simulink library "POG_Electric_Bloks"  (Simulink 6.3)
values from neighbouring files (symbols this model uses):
  al = Tipo(2)    [Flusso_Rotorico_An.m]
  bm = 0.8*N*metri*secondo/rad    (= 0.8)    [architetture_epicicloidale.m]    (also in architetture_epicicloidale_cont.m; architetture_epicicloidale_HEV.m; architetture_epicicloidale_prova.m; architetture_HEV_controllo.m)
  Iw0 = 0*wI0    [architetture_epicicloidale.m]    (also in architetture_epicicloidale_cont.m = wI0; architetture_epicicloidale_HEV.m; architetture_epicicloidale_prova.m; architetture_HEV_controllo.m)
  Jm = 1.6*kg*metri^2    (= 1.6)    [architetture_epicicloidale.m]    (also in architetture_epicicloidale_cont.m; architetture_epicicloidale_HEV.m = 1.64945909552; architetture_epicicloidale_prova.m; architetture_HEV_controllo.m = 0.529459095518)
  Li = 0.1*Henry    (= 0.1)    [architetture_epicicloidale.m]    (also in architetture_epicicloidale_cont.m; architetture_epicicloidale_HEV.m; architetture_epicicloidale_prova.m; architetture_HEV_controllo.m)
  m = 5    [architetture_epicicloidale.m]    (also in architetture_epicicloidale_cont.m; architetture_epicicloidale_HEV.m; architetture_epicicloidale_prova.m; architetture_HEV_controllo.m)
  Mi = 0.08*Henry    (= 0.08)    [architetture_epicicloidale.m]    (also in architetture_epicicloidale_cont.m; architetture_epicicloidale_HEV.m; architetture_epicicloidale_prova.m; architetture_HEV_controllo.m)
  ms = 0.001*secondo    (= 0.001)    [architetture_epicicloidale.m]    (also in architetture_epicicloidale_cont.m; architetture_epicicloidale_HEV.m; architetture_epicicloidale_prova.m; architetture_HEV_controllo.m)
  Nar = 200    [architetture_epicicloidale.m]    (also in architetture_epicicloidale_cont.m; architetture_epicicloidale_HEV.m; architetture_epicicloidale_prova.m; architetture_HEV_controllo.m)
  Nc = 30    [architetture_epicicloidale.m]    (also in architetture_epicicloidale_cont.m; architetture_epicicloidale_HEV.m; architetture_epicicloidale_prova.m; architetture_HEV_controllo.m)
  p = 1    [architetture_epicicloidale.m]    (also in architetture_epicicloidale_cont.m; architetture_epicicloidale_HEV.m; architetture_epicicloidale_prova.m; architetture_HEV_controllo.m)
  Phir = 0.02*Weber    (= 0.02)    [architetture_epicicloidale.m]    (also in architetture_epicicloidale_cont.m; architetture_epicicloidale_HEV.m; architetture_epicicloidale_prova.m; architetture_HEV_controllo.m)
  Ri = 3*Ohm    (= 3)    [architetture_epicicloidale.m]    (also in architetture_epicicloidale_cont.m; architetture_epicicloidale_HEV.m; architetture_epicicloidale_prova.m; architetture_HEV_controllo.m = 0.1)
  Rr = 0.905*m    (= 0.905)    [CVT_New.m]    (also in CVT_New_th.m)
  Star = Si    [architetture_epicicloidale.m]    (also in architetture_epicicloidale_cont.m; architetture_epicicloidale_HEV.m; architetture_epicicloidale_prova.m; architetture_HEV_controllo.m)
  Thm0 = 0    [architetture_epicicloidale.m]    (also in architetture_epicicloidale_cont.m; architetture_epicicloidale_HEV.m; architetture_epicicloidale_prova.m; architetture_HEV_controllo.m)
  Tipo = eval(Flusso(ij).Tipo)    [architetture_epicicloidale.m]    (also in architetture_epicicloidale_cont.m; architetture_epicicloidale_HEV.m; architetture_epicicloidale_prova.m; architetture_HEV_controllo.m)
  Wm0 = 0*Wr_d    (= 0)    [architetture_epicicloidale.m]    (also in architetture_epicicloidale_cont.m = 62.5; architetture_epicicloidale_HEV.m; architetture_epicicloidale_prova.m; architetture_HEV_controllo.m)
undefined symbols (not defined in the file or in its folder): Ib0, Lr, Ls, Lwe, mr, Mr0, Ms0, Msr0, Rs, Rwe
libraries: simulink x10
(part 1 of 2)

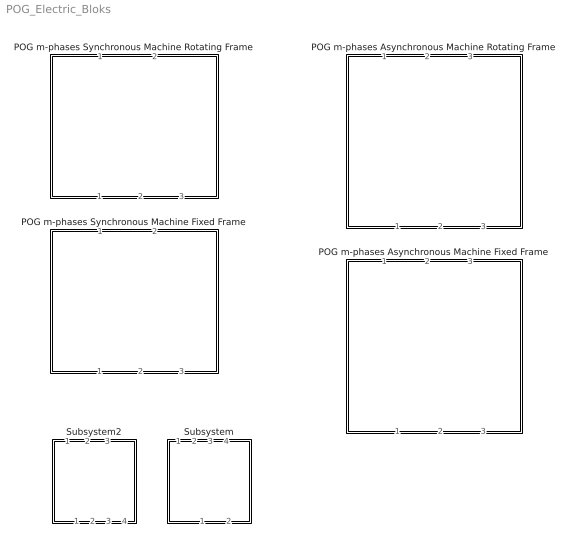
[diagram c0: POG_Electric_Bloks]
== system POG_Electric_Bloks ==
  POG m-phases Asynchronous Machine Fixed Frame : Subsystem  Orientation=down  mask(POG Multi-Phase Motor (Rotating Frame)){Motor_Par=[ms mr], Polar_Par=[p], Electric_S_Par=[Ls Ms0 Rs], Electric_R_Par=[Lr Mr0 Rr], Msr0=Msr0, Mech_Par=[Jm bm], Iniz_Cond=[Wm0; Thm0; Ib0]}
      mask prompts: Motor_Par "Number of phases: [ms, mr] -> [Nr, Nr]"; Polar_Par "Number of polar couples: [p] -> [Nr]"; Electric_S_Par "Stator Parameters: [Ls, Ms0, Rs] -> [Henry, Henry, Ohm]"; Electric_R_Par "Rotor Parameters: [Lr, Mr0, Rr] -> [Henry, Henry, Ohm]"; Msr0 "Mutual Inductance coefficient: [Msr0]-> [Henry]"; Mech_Par "Mechanical Parameters: [Jm, bm] -> [kg*m^2, N m s/rad]"; Iniz_Cond "Initial conditions: [Wm0, Thm0, Ib0] -> [rad/s, rad, A]"
      mask help: Multi-Phase Asynchronous Motor: [ms,mr] = Number of stator and rotor phases; [p] = Number of polar couples; [Ls, Ms0, Rs] = Self inductance, Mutual inductance and Resistance of each stator phase (p=1); [Lr, Mr0, Rr] = Self inductance, Mutual inductance and Resistance of each rotor phase (p=1); [Msr0] = Mutual Inductance coefficient; [Jm, bm] = Inertia momentum, Linear friction coefficient of the rotor; [Wm0, Thm0, Iw0] = Initial conditions on Velocity, Position of the motor and Transformed currents;
      mask init:
      | ms=Motor_Par(1);
      | mr=Motor_Par(2);
      | p =Polar_Par(1);
      | Ls =Electric_S_Par(1);
      | Ms0=Electric_S_Par(2);
      | Rs =Electric_S_Par(3);
      | Lr =Electric_R_Par(1);
      | Mr0=Electric_R_Par(2);
      | Rr =Electric_R_Par(3);
      | Jm=Mech_Par(1);
      | bm=Mech_Par(2);
      | 
      | %%%%%%%%%%%%%%%%%%%%% Initial Conditions
      | if length(Iniz_Cond)<(ms+mr)
      |     Iniz_Cond=[Iniz_Cond; 0*[1:ms+mr-length(Iniz_Cond)]'];
      |     disp('Correction: Iniz_Cond = ...');
      |     disp(Iniz_Cond)
      | end
      | Wm0 = Iniz_Cond(1);
      | Thm0= Iniz_Cond(2);
      | Ib0 = Iniz_Cond(3:ms+mr);
      | 
      | %%%%%%%%%%%%%%%%%%%%%%%%%%%%%%%%%%%%%%%%%%%%%%%%%%%%%%%%%%%%%%%%%%
      | 
      | Ls0=Ls-Ms0;             % stator dispersion self inductance coefficient (p=1)
      | Lse=Ls+(ms-2)*Ms0/2;    % stator transformed self inductance coefficient (p=1)
      | 
      | Lr0=Lr-Mr0;             % rotor dispersion self inductance coefficient (p=1)
      | Lre=Lr+(mr-2)*Mr0/2;    % rotor transformed self inductance coefficient (p=1)
      | 
      | Msre=Msr0*sqrt(ms*mr)/2; % stator-rotor transformed mutual inductance coefficient (p=1)
      | 
      | %%%%%%%%%%%%%%%%%%%%%%%%%%%%%%%%%%%%%%%%%%%%%%%%%%%%%%%%%%%%%%%%%%
      | %%%%%% Trasformazione di coordinate T(s->t)
      | %%%%%%%%%%%%%%%%%%%%%%%%%%%%%%%%%%%%%%%%%%%%%%%%%%%%%%%%%%%%%%%%%%
      | 
      | sTt=[eye(ms) zeros(ms,mr)];
      | 
      | %%%%%%%%%%%%%%%%%%%%%%%%%%%%%%%%%%%%%%%%%%%%%%%%%%%%%%%%%%%%%%%%%%
      | %%%%%% Trasformazione di coordinate T(t->b)
      | %%%%%%%%%%%%%%%%%%%%%%%%%%%%%%%%%%%%%%%%%%%%%%%%%%%%%%%%%%%%%%%%%%
      | 
      | tTb=zeros(ms+mr,ms+mr-2);   
      | %
      | %%%%%%%%%%%%%%%%%%%%%%%%%%%%%%%%%%%%%%%%%%%%%%
      | T_b_Concordia = zeros(ms,ms-1);
      | w = 2*pi/ms;
      | for ii = [1:ms/2]
      |     for jj = [0:ms-1]
      |         T_b_Concordia(jj+1,2*ii-1) = cos((2*ii-1)*w*jj);
      |         T_b_Concordia(jj+1,2*ii  ) = sin((2*ii-1)*w*jj);
      |     end
      | end
      | tTb(1:ms,1:ms-1)=sqrt(2/ms)*T_b_Concordia;       
      | %
      | %%%%%%%%%%%%%%%%%%%%%%%%%%%%%%%%%%%%%%%%%%%%%%
      | T_b_Concordia = zeros(mr,mr-1);
      | w = 2*pi/mr;
      | for ii = [1:mr/2]
      |     for jj = [0:mr-1]
      |         T_b_Concordia(jj+1,2*ii-1) = cos((2*ii-1)*w*jj);
      |         T_b_Concordia(jj+1,2*ii  ) = sin((2*ii-1)*w*jj);
      |     end
      | end
      | tTb(ms+1:ms+mr,ms:ms+mr-2)=sqrt(2/mr)*T_b_Concordia;       
      | 
      | %%%%%%%%%%%%%%%%%%%%%%%%%%%%%%%%%%%%%%%%%%%%%%%%%%%%%%%%%%%%%%%%%%
      | %%%%%% Matrici LMbe e Rbe nel frame ruotante w
      | %%%%%%%%%%%%%%%%%%%%%%%%%%%%%%%%%%%%%%%%%%%%%%%%%%%%%%%%%%%%%%%%%%
      | 
      | LMbe=zeros(ms+mr-2);            % Matrice LMbe
      | LMbe(1:2,1:2)=eye(2)*Lse;        
      | LMbe(3:ms-1,3:ms-1)=eye(ms-3)*Ls0;        
      | LMbe(ms:ms+1,ms:ms+1)=eye(2)*Lre;        
      | LMbe(ms+2:ms+mr-2,ms+2:ms+mr-2)=eye(mr-3)*Lr0;        
      | LMbe=p*LMbe;
      | 
      | Mbe=zeros(ms+mr-2);            % Matrice Mbe
      | Mbe(1:2,ms:ms+1)=eye(2);        
      | Mbe(ms:ms+1,1:2)=eye(2);        
      | 
      | JKb=zeros(ms+mr-2);            % Matrice JKb             
      | JKb(2,1)=-1;  
      | JKb(1,2)=1;  
      | JKb(ms+1,ms)=1;  
      | JKb(ms,ms+1)=-1;  
      | 
      | Lbe=LMbe+Mbe*cos(p*Thm0)-JKb*sin(p*Thm0);
      | 
      | Rbe=zeros(ms+mr-2);            % Matrice Rbe
      | Rbe(1:ms-1,1:ms-1)=eye(ms-1)*Rs;        
      | Rbe(ms:ms+mr-2,ms:ms+mr-2)=eye(mr-1)*Rr;        
      | 
      | %%%%%%%%%%%%%%%%%%%%%%%%%%%%%%%%%%%%%%%%%%%%%%%%%%%%%%%%%%%%%%%%%%
  POG m-phases Asynchronous Machine Rotating Frame : Subsystem  Orientation=down  mask(POG Multi-Phase Motor (Rotating Frame)){Motor_Par=[ms mr], Polar_Par=[p], Electric_S_Par=[Ls Ms0 Rs], Electric_R_Par=[Lr Mr0 Rr], Msr0=Msr0, Mech_Par=[Jm bm], Iniz_Cond=[Wm0; Thm0; Iw0]}
      mask prompts: Motor_Par "Number of phases: [ms, mr] -> [Nr, Nr]"; Polar_Par "Number of polar couples: [p] -> [Nr]"; Electric_S_Par "Stator Parameters: [Ls, Ms0, Rs] -> [Henry, Henry, Ohm]"; Electric_R_Par "Rotor Parameters: [Lr, Mr0, Rr] -> [Henry, Henry, Ohm]"; Msr0 "Mutual Inductance coefficient: [Msr0]-> [Henry]"; Mech_Par "Mechanical Parameters: [Jm, bm] -> [kg*m^2, N m s/rad]"; Iniz_Cond "Initial conditions: [Wm0, Thm0, Iw0] -> [rad/s, rad, A]"
      mask help: Multi-Phase Asynchronous Motor: [ms,mr] = Number of stator and rotor phases; [p] = Number of polar couples; [Ls, Ms0, Rs] = Self inductance, Mutual inductance and Resistance of each stator phase (p=1); [Lr, Mr0, Rr] = Self inductance, Mutual inductance and Resistance of each rotor phase (p=1); [Msr0] = Mutual Inductance coefficient; [Jm, bm] = Inertia momentum, Linear friction coefficient of the rotor; [Wm0, Thm0, Iw0] = Initial conditions on Velocity, Position of the motor and Transformed currents;
      mask init:
      | ms=Motor_Par(1);
      | mr=Motor_Par(2);
      | p =Polar_Par(1);
      | Ls =Electric_S_Par(1);
      | Ms0=Electric_S_Par(2);
      | Rs =Electric_S_Par(3);
      | Lr =Electric_R_Par(1);
      | Mr0=Electric_R_Par(2);
      | Rr =Electric_R_Par(3);
      | Jm=Mech_Par(1);
      | bm=Mech_Par(2);
      | 
      | %%%%%%%%%%%%%%%%%%%%% Initial Conditions
      | if length(Iniz_Cond)<(ms+mr)
      |     Iniz_Cond=[Iniz_Cond; 0*[1:ms+mr-length(Iniz_Cond)]'];
      |     disp('Correction: Iniz_Cond = ...');
      |     disp(Iniz_Cond)
      | end
      | Wm0 = Iniz_Cond(1);
      | Thm0= Iniz_Cond(2);
      | Iw0 = Iniz_Cond(3:ms+mr);
      | 
      | Ls0=Ls-Ms0;             % stator dispersion self inductance coefficient (p=1)
      | Lse=Ls+(ms-2)*Ms0/2;    % stator transformed self inductance coefficient (p=1)
      | 
      | Lr0=Lr-Mr0;             % rotor dispersion self inductance coefficient (p=1)
      | Lre=Lr+(mr-2)*Mr0/2;    % rotor transformed self inductance coefficient (p=1)
      | 
      | Msre=Msr0*sqrt(ms*mr)/2; % stator-rotor transformed mutual inductance coefficient (p=1)
      | 
      | %%%%%%%%%%%%%%%%%%%%%%%%%%%%%%%%%%%%%%%%%%%%%%%%%%%%%%%%%%%%%%%%%%
      | %%%%%% Trasformazione di coordinate T(s->t)
      | %%%%%%%%%%%%%%%%%%%%%%%%%%%%%%%%%%%%%%%%%%%%%%%%%%%%%%%%%%%%%%%%%%
      | 
      | sTt=[eye(ms) zeros(ms,mr)];
      | 
      | %%%%%%%%%%%%%%%%%%%%%%%%%%%%%%%%%%%%%%%%%%%%%%%%%%%%%%%%%%%%%%%%%%
      | %%%%%% Trasformazione di coordinate T(t->b)
      | %%%%%%%%%%%%%%%%%%%%%%%%%%%%%%%%%%%%%%%%%%%%%%%%%%%%%%%%%%%%%%%%%%
      | 
      | tTb=zeros(ms+mr,ms+mr-2);   
      | %
      | %%%%%%%%%%%%%%%%%%%%%%%%%%%%%%%%%%%%%%%%%%%%%%
      | T_b_Concordia = zeros(ms,ms-1);
      | w = 2*pi/ms;
      | for i = [1:ms/2]
      |     for j = [0:ms-1]
      |         T_b_Concordia(j+1,2*i-1) = cos((2*i-1)*w*j);
      |         T_b_Concordia(j+1,2*i  ) = sin((2*i-1)*w*j);
      |     end
      | end
      | tTb(1:ms,1:ms-1)=sqrt(2/ms)*T_b_Concordia;       
      | %
      | %%%%%%%%%%%%%%%%%%%%%%%%%%%%%%%%%%%%%%%%%%%%%%
      | T_b_Concordia = zeros(mr,mr-1);
      | w = 2*pi/mr;
      | for i = [1:mr/2]
      |     for j = [0:mr-1]
      |         T_b_Concordia(j+1,2*i-1) = cos((2*i-1)*w*j);
      |         T_b_Concordia(j+1,2*i  ) = sin((2*i-1)*w*j);
      |     end
      | end
      | tTb(ms+1:ms+mr,ms:ms+mr-2)=sqrt(2/mr)*T_b_Concordia;       
      | 
      | %%%%%%%%%%%%%%%%%%%%%%%%%%%%%%%%%%%%%%%%%%%%%%%%%%%%%%%%%%%%%%%%%%
      | %%%%%% Trasformazione di coordinate T(b->w)
      | %%%%%%%%%%%%%%%%%%%%%%%%%%%%%%%%%%%%%%%%%%%%%%%%%%%%%%%%%%%%%%%%%%
      | 
      | MKs=zeros(ms+mr-2);             % Matrice MKs
      | MKs(1:2,1:2)=eye(2);  
      | 
      | MKr=zeros(ms+mr-2);             % Matrice MKr             
      | MKr(ms:ms+1,ms:ms+1)=eye(2);  
      | 
      | I_m=eye(ms+mr-2);               % Matrice I_m
      | 
      | Jsr= zeros(ms+mr-2);            % Matrice Jsr
      | for j=[2:2:ms+mr-2]
      |     Jsr(j,j-1)= 1;
      |     Jsr(j-1,j)=-1;
      | end
      | 
      | %%%%%%%%%%%%%%%%%%%%%%%%%%%%%%%%%%%%%%%%%%%%%%%%%%%%%%%%%%%%%%%%%%
      | %%%%%% Matrici Lw_e e Rw_e nel frame ruotante w
      | %%%%%%%%%%%%%%%%%%%%%%%%%%%%%%%%%%%%%%%%%%%%%%%%%%%%%%%%%%%%%%%%%%
      | 
      | Lwe=zeros(ms+mr-2);            % Matrice Lw_e
      | Lwe(1:2,1:2)=eye(2)*Lse;        
      | Lwe(3:ms-1,3:ms-1)=eye(ms-3)*Ls0;        
      | Lwe(ms:ms+1,ms:ms+1)=eye(2)*Lre;        
      | Lwe(ms+2:ms+mr-2,ms+2:ms+mr-2)=eye(mr-3)*Lr0;        
      | Lwe(1:2,ms:ms+1)=eye(2)*Msre;        
      | Lwe(ms:ms+1,1:2)=eye(2)*Msre;        
      | Lwe=p*Lwe;
      | 
      | 
      | Rwe=zeros(ms+mr-2);            % Matrice Rw_e
      | Rwe(1:ms-1,1:ms-1)=eye(ms-1)*Rs;        
      | Rwe(ms:ms+mr-2,ms:ms+mr-2)=eye(mr-1)*Rr;        
      | 
      | Ks=zeros(ms+mr-2,1);           % Matrice Ks
      | Ks(1:2)=[1;1];  
      | 
      | Kr=zeros(ms+mr-2,1);           % Matrice Kr             
      | Kr(ms:ms+1)=[1;1];  
      | 
      | JK=zeros(ms+mr-2);            % Matrice JKe             
      | JK(ms+1,1)=1;  
      | JK(ms,2)=-1;  
      | JK(1,ms+1)=1;  
      | JK(2,ms)=-1;  
      | JKe=-p^2*Msre*JK/2;
      | JFe=p*Msre*JK/2;
      | 
      | %%%%%%%%%%%%%%%%%%%%%%%%%%%%%%%%%%%%%%%%%%%%%%%%%%%%%%%%%%%%%%%%%%
  POG m-phases Synchronous Machine Fixed Frame : Subsystem  Orientation=down  mask(POG Multi-Phase Motor (Fixed Frame)){Motor_Par=[m p], Phase_Par=[Nc Star], Electric_Par=[Ri Li Mi], Mech_Par=[Jm bm], Plux_Par=[Phir Nar], Iniz_Cond=[Wm0; Thm0; Iw0], TipoFlux=Fourier defined, Tipo=Tipo, alfa=al, degree=6, TipoF=Tipo}
      mask prompts: Motor_Par "Number of phases, Number of polar couples: [m, p] -> [Nr, Nr]"; Phase_Par "Number of coils, Star connected?: [Nc, Star] -> [Nr, (True, False)]"; Electric_Par "Electric Parameters: [Ri, Li, Mi] -> [Henry, Henry, Ohm]"; Mech_Par "Mechanical Parameters: [Jm, bm] -> [kg*m^2, N m s/rad]"; Plux_Par "Maximum value of the rotor flux, Number of Fourier harmonics: [Phir, Nar] -> [W, Nr]"; Iniz_Cond "Initial conditions: [Wm0, Thm0, It0] -> [rad/s, rad, A]"; TipoFlux "Type of Rotor Flux"; Tipo "Type defined by user: Tipo -> [Nr,alfa,degree]"; alfa "Flux function parameter: alfa -> [0, pi/2]:"; degree "Degree of the polinomial flux function:"; TipoF "Components of the Fourier series: [9, Nmax, CompAi] -> [9, Nr, a0, a1, ..., aNr]"
      mask help: Multi-Phase Permanent Magnet Synchronous Motor: [m, p] = Number of motor phases, Polar couples; [Nc, Star] = Number of coils per phase, Type of phase connection; [Ri, Li, Mi] = Resistance, Self inductance, Mutual inductance of each phase; [Jm, bm] = Inertia momentum, Friction coefficient of the rotor; [Phir, Nar] = Maximum value of the rotor flux, Number of Fourier harmonics; [Wm0, Thm0, Iw0] = Initial conditions on Velocity, Position of the motor and Currents; Type of Rotor Flux (Tipo): Trapezoidal [1,alfa]; Triangular [1, 0]; Squared wave [2]; Sinusoidal [3]; Cosinusoidally connected [4,alfa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
      mask init:
      | m=Motor_Par(1);
      | p=Motor_Par(2);
      | Nc=Phase_Par(1);
      | Star=Phase_Par(2);
      | Ri=Electric_Par(1);
      | Li=Electric_Par(2);
      | Mi=Electric_Par(3);
      | Jm=Mech_Par(1);
      | bm=Mech_Par(2);
      | Phir=Plux_Par(1);
      | Nar=Plux_Par(2);
      | 
      | %%%%%%%%%%%%%%%%%%%%% Initial Conditions
      | if length(Iniz_Cond)<(m+2-Star)
      |     Iniz_Cond=[Iniz_Cond 0*[1:m+2-Star-length(Iniz_Cond)]];
      |     disp('Correction: Iniz_Cond = ...');
      |     disp(Iniz_Cond)
      | end
      | Wm0 = Iniz_Cond(1);
      | Thm0= Iniz_Cond(2);
      | Ibt0 = Iniz_Cond(3:m+2-Star);
      | 
      | %%%%%%%%%%%%%%%%%%%%%%%%%%%%
      | FluxName(1)=struct('Nome','Trapezoidal');
      | FluxName(2)=struct('Nome','Squared wave');
      | FluxName(3)=struct('Nome','Sinusoidal');
      | FluxName(4)=struct('Nome','Cosinusoidally connected');
      | FluxName(5)=struct('Nome','Sinusoidally connected');
      | FluxName(6)=struct('Nome','Polynomial even');
      | FluxName(7)=struct('Nome','Polynomial odd');
      | FluxName(8)=struct('Nome','Trapezoidal if derived');
      | FluxName(9)=struct('Nome','Fourier defined');
      | 
      | switch TipoFlux
      |     case 'User defined',
      |     case 'Trapezoidal'
      |         if alfa<0, alfa=0; disp('Correction: alfa = 0'); end
      |         if alfa>pi/2, alfa=pi/2; disp('Correction: alfa = pi/2'); end
      |         Tipo = [1,alfa];
      |     case 'Triangular'
      |         Tipo = [1,  0];
      |     case 'Squared wave'
      |         Tipo = [2];
      |     case 'Sinusoidal'
      |         Tipo = [3];
      |     case 'Cosinusoidally connected'
      |         if alfa<0, alfa=0; disp('Correction: alfa = 0'); end
      |         if alfa>pi/2, alfa=pi/2; disp('Correction: alfa = pi/2'); end
      |         Tipo = [4,alfa];
      |     case 'Sinusoidally connected'
      |         if alfa<0, alfa=0; disp('Correction: alfa = 0'); end
      |         if alfa>pi/2, alfa=pi/2; disp('Correction: alfa = pi/2'); end
      |         Tipo = [5,alfa];
      |     case 'Polynomial even'
      |         if alfa<0, alfa=0; disp('Correction: alfa = 0'); end
      |         if alfa>pi/2, alfa=pi/2; disp('Correction: alfa = pi/2'); end
      |         if rem(degree)==1, 
      |             degree=degree-1; 
      |             disp(['Correction: degree = ' num2str(degree)]); 
      |         end
      |         if degree<2
      |             degree=2; 
      |             disp(['Correction: degree = ' num2str(degree)]); 
      |         end            
      |         Tipo = [6,alfa,degree];
      |     case 'Polynomial odd'
      |         if alfa<0, alfa=0; disp('Correction: alfa = 0'); end
      |         if alfa>pi/2, alfa=pi/2; disp('Correction: alfa = pi/2'); end
      |         if rem(degree)==0, 
      |             degree=degree-1; 
      |             disp(['Correction: degree = ' num2str(degree)]); 
      |         end
      |         if degree<1
      |             degree=1; 
      |             disp(['Correction: degree = ' num2str(degree)]); 
      |         end            
      |         Tipo = [7,alfa,degree];
      |     case 'Trapezoidal if derived'
      |         Tipo = [8,alfa];
      |         if alfa<0, alfa=0; disp('Correction: alfa = 0'); end
      |         if alfa>pi/2, alfa=pi/2; disp('Correction: alfa = pi/2'); end
      |     case 'Fourier defined'
      |         if TipoF(1)~=9
      |             disp('Correction: NrType = 9 (Fourier defined)')
      |             TipoF(1)=9;
      |         end
      |         if length(TipoF)<2
      |             TipoF(2)=m;
      |             disp('Correction: Fourier defined -> TipoF = ...');
      |             disp(TipoF)
      |         end
      |         if TipoF(2)<m,
      |             TipoF(2)=m;
      |             disp('Correction: Fourier defined -> Nas = m');
      |         end
      |         if length(TipoF)<(TipoF(2)+3)
      |             TipoF=[TipoF 0*[1:TipoF(2)+3-length(TipoF)]];
      |             disp('Correction: Fourier defined -> TipoF = ...'); 
      |             disp(TipoF)
      |         end
      |         Tipo = TipoF;   % [9,Nmax,CompAi]
      |     otherwise,
      |         disp('Flux type not correct')
      |         return
      | end
      | 
      | switch TipoFlux
      |     case 'User defined',
      |         disp(['The rotor flux is ''''' FluxName(Tipo(1)).Nome ''''' (Us. Def.)'])
      |     otherwise,
      |         disp(['The rotor flux is ''''' TipoFlux ''''''])
      | end
      | 
      | 
      | %%%%%%%%%%%%%%%%%%%%%%%%%%%%%
      | tTb=T_b_Concordia(m);       %%% Trasformazione "T(b->t)": matrice tTb;
      | 
      | MLb=p*eye(m)*(Li-Mi);       %%% Auto and mutual inductance matrix MLb 
      | MLb(1,1)=p*(Li+(m-2)*Mi/2); %%% defined in the rotating frame
      | MLb(2,2)=p*(Li+(m-2)*Mi/2);
      | 
      | MR = p*Ri*eye(m);           %%% Resistance matrice MR defined in the rotating frame
      | %
      | Phic = p*Nc*Phir;           %%% Maximum value of the concatenated flux;
      | %
      | if Nar<m,
      |     Nar=m;
      |     disp('Correction: Nar = m');
      | end
      | if Star                     %%% Reduction of the system matrices if Star is True
      |     tTabc=tTb(:,[1:m-1]);
      |     MLabc=MLb([1:m-1],[1:m-1]);
      |     MRabc=MR([1:m-1],[1:m-1]);
      |     Ibt0=MLabc*Ibt0;
      | else
      |     tTabc=eye(m);
      |     MLabc=tTb*MLb*tTb';
      |     MRabc=tTb*MR*tTb';
      |     Ibt0=MLabc*tTabc'*Ibt0;
      | end
      | Sfasa  = -2*pi*[0:m-1]'/m;   % Matrice di sfasamento
      | LkUpT_in=[-1:0.0001:1]*2*pi;
      | LkUpT_out=0*LkUpT_in;
      | for n=[1:2:Nar]
      |     LkUpT_out=LkUpT_out-Flusso_Rotorico_An(Tipo,n)*n*sin(n*LkUpT_in);
      | end
      | LkUpT_out=p*Phic*LkUpT_out;
  POG m-phases Synchronous Machine Rotating Frame : Subsystem  Orientation=down  mask(POG Multi-Phase Motor (Rotating Frame)){Motor_Par=[m p], Phase_Par=[Nc Star], Electric_Par=[Ri Li Mi], Mech_Par=[Jm bm], Plux_Par=[Phir Nar], Iniz_Cond=[Wm0; Thm0; Iw0], TipoFlux=Fourier defined, Tipo=Tipo, alfa=al, degree=6, TipoF=Tipo}
      mask prompts: Motor_Par "Number of phases, Number of polar couples: [m, p] -> [Nr, Nr]"; Phase_Par "Number of coils, Star connected?: [Nc, Star] -> [Nr, (True, False)]"; Electric_Par "Electric Parameters: [Ri, Li, Mi] -> [Henry, Henry, Ohm]"; Mech_Par "Mechanical Parameters: [Jm, bm] -> [kg*m^2, N m s/rad]"; Plux_Par "Maximum value of the rotor flux, Number of Fourier harmonics: [Phir, Nar] -> [W, Nr]"; Iniz_Cond "Initial conditions: [Wm0, Thm0, Iw0] -> [rad/s, rad, A]"; TipoFlux "Type of Rotor Flux"; Tipo "Type defined by user: Tipo -> [Nr,alfa,degree]"; alfa "Flux function parameter: alfa -> [0, pi/2]:"; degree "Degree of the polinomial flux function:"; TipoF "Components of the Fourier series: [9, Nmax, CompAi] -> [9, Nr, a0, a1, ..., aNr]"
      mask help: Multi-Phase Permanent Magnet Synchronous Motor: [m, p] = Number of motor phases, Polar couples; [Nc, Star] = Number of coils per phase, Type of phase connection; [Ri, Li, Mi] = Resistance, Self inductance, Mutual inductance of each phase; [Jm, bm] = Inertia momentum, Friction coefficient of the rotor; [Phir, Nar] = Maximum value of the rotor flux, Number of Fourier harmonics; [Wm0, Thm0, Iw0] = Initial conditions on Velocity, Position of the motor and Currents; Type of Rotor Flux (Tipo): Trapezoidal [1,alfa]; Triangular [1, 0]; Squared wave [2]; Sinusoidal [3]; Cosinusoidally connected [4,alfa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
      mask init:
      | m=Motor_Par(1);
      | p=Motor_Par(2);
      | Nc=Phase_Par(1);
      | Star=Phase_Par(2);
      | Ri=Electric_Par(1);
      | Li=Electric_Par(2);
      | Mi=Electric_Par(3);
      | Jm=Mech_Par(1);
      | bm=Mech_Par(2);
      | Phir=Plux_Par(1);
      | Nar=Plux_Par(2);
      | 
      | %%%%%%%%%%%%%%%%%%%%% Initial Conditions
      | if length(Iniz_Cond)<(m+2-Star)
      |     Iniz_Cond=[Iniz_Cond 0*[1:m+2-Star-length(Iniz_Cond)]];
      |     disp('Correction: Iniz_Cond = ...');
      |     disp(Iniz_Cond)
      | end
      | Wm0 = Iniz_Cond(1);
      | Thm0= Iniz_Cond(2);
      | Iw0 = Iniz_Cond(3:m+2-Star);
      | 
      | %%%%%%%%%%%%%%%%%%%%%%%%%%%%
      | FluxName(1)=struct('Nome','Trapezoidal');
      | FluxName(2)=struct('Nome','Squared wave');
      | FluxName(3)=struct('Nome','Sinusoidal');
      | FluxName(4)=struct('Nome','Cosinusoidally connected');
      | FluxName(5)=struct('Nome','Sinusoidally connected');
      | FluxName(6)=struct('Nome','Polynomial even');
      | FluxName(7)=struct('Nome','Polynomial odd');
      | FluxName(8)=struct('Nome','Trapezoidal if derived');
      | FluxName(9)=struct('Nome','Fourier defined');
      | 
      | switch TipoFlux
      |     case 'User defined',
      |     case 'Trapezoidal'
      |         if alfa<0, alfa=0; disp('Correction: alfa = 0'); end
      |         if alfa>pi/2, alfa=pi/2; disp('Correction: alfa = pi/2'); end
      |         Tipo = [1,alfa];
      |     case 'Triangular'
      |         Tipo = [1,  0];
      |     case 'Squared wave'
      |         Tipo = [2];
      |     case 'Sinusoidal'
      |         Tipo = [3];
      |     case 'Cosinusoidally connected'
      |         if alfa<0, alfa=0; disp('Correction: alfa = 0'); end
      |         if alfa>pi/2, alfa=pi/2; disp('Correction: alfa = pi/2'); end
      |         Tipo = [4,alfa];
      |     case 'Sinusoidally connected'
      |         if alfa<0, alfa=0; disp('Correction: alfa = 0'); end
      |         if alfa>pi/2, alfa=pi/2; disp('Correction: alfa = pi/2'); end
      |         Tipo = [5,alfa];
      |     case 'Polynomial even'
      |         if alfa<0, alfa=0; disp('Correction: alfa = 0'); end
      |         if alfa>pi/2, alfa=pi/2; disp('Correction: alfa = pi/2'); end
      |         if rem(degree)==1, 
      |             degree=degree-1; 
      |             disp(['Correction: degree = ' num2str(degree)]); 
      |         end
      |         if degree<2
      |             degree=2; 
      |             disp(['Correction: degree = ' num2str(degree)]); 
      |         end            
      |         Tipo = [6,alfa,degree];
      |     case 'Polynomial odd'
      |         if alfa<0, alfa=0; disp('Correction: alfa = 0'); end
      |         if alfa>pi/2, alfa=pi/2; disp('Correction: alfa = pi/2'); end
      |         if rem(degree)==0, 
      |             degree=degree-1; 
      |             disp(['Correction: degree = ' num2str(degree)]); 
      |         end
      |         if degree<1
      |             degree=1; 
      |             disp(['Correction: degree = ' num2str(degree)]); 
      |         end            
      |         Tipo = [7,alfa,degree];
      |     case 'Trapezoidal if derived'
      |         Tipo = [8,alfa];
      |         if alfa<0, alfa=0; disp('Correction: alfa = 0'); end
      |         if alfa>pi/2, alfa=pi/2; disp('Correction: alfa = pi/2'); end
      |     case 'Fourier defined'
      |         if TipoF(1)~=9
      |             disp('Correction: NrType = 9 (Fourier defined)')
      |             TipoF(1)=9;
      |         end
      |         if length(TipoF)<2
      |             TipoF(2)=m;
      |             disp('Correction: Fourier defined -> TipoF = ...');
      |             disp(TipoF)
      |         end
      |         if TipoF(2)<m,
      |             TipoF(2)=m;
      |             disp('Correction: Fourier defined -> Nas = m');
      |         end
      |         if length(TipoF)<(TipoF(2)+3)
      |             TipoF=[TipoF 0*[1:TipoF(2)+3-length(TipoF)]];
      |             disp('Correction: Fourier defined -> TipoF = ...'); 
      |             disp(TipoF)
      |         end
      |         Tipo = TipoF;   % [9,Nmax,CompAi]
      |     otherwise,
      |         disp('Flux type not correct')
      |         return
      | end
      | 
      | switch TipoFlux
      |     case 'User defined',
      |         disp(['The rotor flux is ''''' FluxName(Tipo(1)).Nome ''''' (Us. Def.)'])
      |     otherwise,
      |         disp(['The rotor flux is ''''' TipoFlux ''''''])
      | end
      | 
      | 
      | %%%%%%%%%%%%%%%%%%%%%%%%%%%%%
      | tTb=T_b_Concordia(m);       %%% Trasformazione "T(b->t)": matrice tTb;
      | 
      | MKr= zeros(m);              %%% Trasformazione "T(b->w)": matrici MKr, Jr e I_m;
      | for j=[1:2:m-1]
      |     MKr(j,j)= j;  MKr(j+1,j+1)= j;
      | end
      | Jr= zeros(m);
      | for j=[2:2:m]
      |     Jr(j-1,j)= 1;  Jr(j,j-1)=-1;
      | end
      | I_m=eye(m);
      | 
      | MLb=p*eye(m)*(Li-Mi);       %%% Auto and mutual inductance matrix MLb 
      | MLb(1,1)=p*(Li+(m-2)*Mi/2); %%% defined in the rotating frame
      | MLb(2,2)=p*(Li+(m-2)*Mi/2);
      | 
      | MR = p*Ri*eye(m);           %%% Resistance matrice MR defined in the rotating frame
      | %
      | Kr= zeros(m,1);             %%% Matrix Kr for the energy redistribution "j*w*L"
      | for j=[1:2:m-1]
      |     Kr(j)= j;  Kr(j+1)= j;
      | end
      | %
      | Phic = p*Nc*Phir;           %%% Maximum value of the concatenated flux;
      | %
      | if Nar<m,
      |     Nar=m;
      |     disp('Correction: Nar = m');
      | end
      | N_2m_2m=[0:2*m:Nar]';       %%% Matrices N_2m_2m, N_m_2m, An_sin, An_sin, M_gira
      | N_m_2m =[m:2*m:Nar]';       %%% for the computation of the torque vector "Ktau"
      | An_sin=zeros((m-1)/2,max(size(N_2m_2m)));
      | An_cos=zeros((m-1)/2,max(size(N_2m_2m)));
      | for k=[1:2:m-1]
      |     An_piu_k = Flusso_Rotorico_An(Tipo,N_2m_2m+k)';
      |     An_men_k = Flusso_Rotorico_An(Tipo,N_2m_2m-k)';
      |     An_sin((k+1)/2,:) = -p*sqrt(m/2)*Phic*(An_piu_k.*(N_2m_2m'+k) + An_men_k.*(N_2m_2m'-k));
      |     An_cos((k+1)/2,:) = -p*sqrt(m/2)*Phic*(An_piu_k.*(N_2m_2m'+k) - An_men_k.*(N_2m_2m'-k));
      | end
      | An_m_sin = -p*sqrt(m)*Phic*(Flusso_Rotorico_An(Tipo,N_m_2m)').*N_m_2m';
      | M_gira=eye(m);
      | M_gira=[M_gira(:,1:2:m-1) M_gira(:,2:2:m-1) M_gira(:,m)];
      | %
      | if Star        %%% Reduction of the system matrices if Star is True
      |     tTb=tTb(:,[1:m-1]);
      |     MKr=MKr([1:m-1],[1:m-1]);
      |     Jr=Jr([1:m-1],[1:m-1]);
      |     I_m=eye(m-1);
      |     MLb=MLb([1:m-1],[1:m-1]);
      |     MR=MR([1:m-1],[1:m-1]);
      |     Kr=Kr([1:m-1]);
      |     M_gira=M_gira([1:m-1],:);
      | end
      | %
  Subsystem : Subsystem  Orientation=down
  Subsystem2 : Subsystem  Orientation=down  mask(Dynamic Power Flow){L=Lwe, R=Rwe}
      mask prompts: L "The dynamic element [L, C, J, ...]"; R "The Dissipative element [R,G, b,...]"
      mask help: Calcola il bilancio energetico di un elemento dinamico "lineare" avente (v1,v2) come porta energetica di ingresso e (v3,v2) come porta energetica di uscita. L'elemento dinamico interno genera la variabile di potenza v2. Parametri: L Elemento dinamico che accumula energia: equazione costitutiva q2=L*v2. R Elemento statico che dissipa energia: equazione costitutiva vr=R*v2. Fornisce in uscita le seguenti variabili: DP Differenza fra la Potenza in ingresso e quella in uscita; Pd Potenza dissipata all'interno dell'elemento; Ea Energia accumulata all'interno dell'elemento; DE Differenza Energetica 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

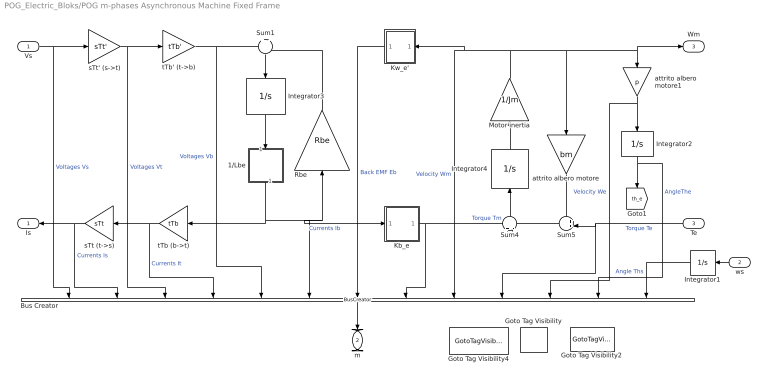
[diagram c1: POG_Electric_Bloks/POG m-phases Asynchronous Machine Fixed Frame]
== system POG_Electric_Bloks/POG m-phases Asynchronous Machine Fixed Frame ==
  Vs : Inport
  ws : Inport  Orientation=left  Port=2
  Te : Inport  Orientation=left  Port=3
  1/Lbe : Subsystem  Orientation=down
  Bus Creator : BusCreator  Orientation=down  Inputs=13
  Goto Tag Visibility : GotoTagVisibility
  Goto Tag Visibility2 : GotoTagVisibility
  Goto Tag Visibility4 : GotoTagVisibility
  Integrator1 : Integrator  Orientation=left
  Integrator2 : Integrator  Orientation=down  InitialCondition=Thm0*p
  Integrator3 : Integrator  Orientation=down  InitialCondition=Lbe*Ib0
  Integrator4 : Integrator  Orientation=up  InitialCondition=Wm0*Jm
  Kb_e : Subsystem
  Kw_e' : Subsystem  Orientation=left
  Motor inertia : Gain  Orientation=up  Gain=1/Jm
  Rbe : Gain  Orientation=up  Gain=Rbe  Multiplication=Matrix(K*u) (u vector)
  Sum1 : Sum  Orientation=down  Inputs=+|-
  Sum4 : Sum  Orientation=up  Inputs=+|-
  Sum5 : Sum  Orientation=left  Inputs=++|
  attrito albero motore : Gain  Orientation=down  Gain=bm
  attrito albero motore1 : Gain  Orientation=down  Gain=p
  sTt (t->s) : Gain  Orientation=left  Gain=sTt  Multiplication=Matrix(K*u) (u vector)
  sTt' (s->t) : Gain  Gain=sTt'  Multiplication=Matrix(K*u) (u vector)
  tTb (b->t) : Gain  Orientation=left  Gain=tTb  Multiplication=Matrix(K*u) (u vector)
  tTb' (t->b) : Gain  Gain=tTb'  Multiplication=Matrix(K*u) (u vector)
  Is : Outport  Orientation=left
  m : Outport  Orientation=down  Port=2
  Wm : Outport  Port=3
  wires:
  Integrator1/1 -> Bus Creator/13  "Angle Ths"
  ws/1 -> Integrator1/1
  Kw_e'/1(Eb) -> Bus Creator/7  "Back EMF Eb"
  Rbe/1 -> Sum1/2
  Bus Creator/1 -> m/1
  tTb (b->t)/1 -> Bus Creator/4, sTt (t->s)/1  "Currents It"
  Te/1 -> Bus Creator/10, Sum5/2  "Torque Te"
  Vs/1 -> Bus Creator/1, sTt' (s->t)/1  "Voltages Vs"
  attrito albero motore/1 -> Sum5/1
  Motor inertia/1 -> Bus Creator/9, Kw_e'/1(Wm), attrito albero motore/1, Wm/1, attrito albero motore1/1  "Velocity Wm"
  Integrator4/1 -> Motor inertia/1
  Sum4/1 -> Integrator4/1
  Kb_e/1(Tm) -> Bus Creator/8, Sum4/1  "Torque Tm"
  1/Lbe/1(Ib) -> tTb (b->t)/1, Bus Creator/6, Kb_e/1(Ib), Rbe/1  "Currents Ib"
  Integrator3/1 -> 1/Lbe/1(Phib)
  Sum1/1 -> Integrator3/1
  Integrator2/1 -> Bus Creator/12, [th_e]  "AngleThe"
  attrito albero motore1/1 -> Bus Creator/11, Integrator2/1  "Velocity We"
  tTb' (t->b)/1 -> Sum1/1, Bus Creator/5  "Voltages Vb"
  Sum5/1 -> Sum4/2
  sTt (t->s)/1 -> Bus Creator/2, Is/1  "Currents Is"
  sTt' (s->t)/1 -> Bus Creator/3, tTb' (t->b)/1  "Voltages Vt"

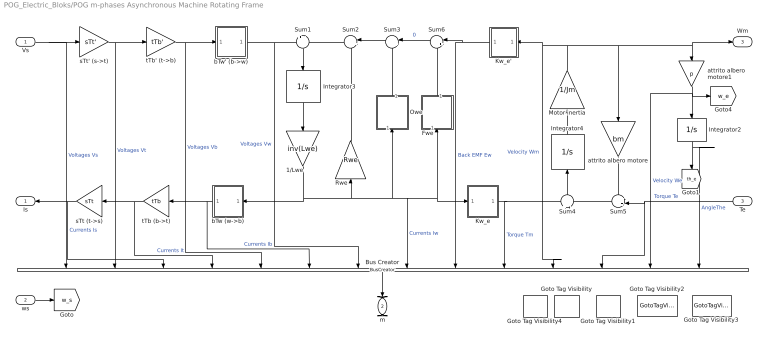
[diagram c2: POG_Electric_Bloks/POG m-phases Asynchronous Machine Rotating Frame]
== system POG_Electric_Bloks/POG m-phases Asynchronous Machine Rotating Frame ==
  Vs : Inport
  ws : Inport  Port=2
  Te : Inport  Orientation=left  Port=3
  1/Lwe : Gain  Orientation=down  Gain=inv(Lwe)  Multiplication=Matrix(K*u) (u vector)
  Bus Creator : BusCreator  Orientation=down  Inputs=14
  Fwe : Subsystem  Orientation=up
  Goto Tag Visibility{,1..4} (5 alike) : GotoTagVisibility
  Integrator2 : Integrator  Orientation=down  InitialCondition=Thm0*p
  Integrator3 : Integrator  Orientation=down  InitialCondition=Lwe*Iw0
  Integrator4 : Integrator  Orientation=up  InitialCondition=Wm0*Jm
  Kw_e : Subsystem
  Kw_e' : Subsystem  Orientation=left
  Motor inertia : Gain  Orientation=up  Gain=1/Jm
  Owe : Subsystem  Orientation=up
  Rwe : Gain  Orientation=up  Gain=Rwe  Multiplication=Matrix(K*u) (u vector)
  Sum1 : Sum  Orientation=down  Inputs=+|-
  Sum2 : Sum  Orientation=left  Inputs=|++
  Sum3 : Sum  Orientation=left  Inputs=|++
  Sum4 : Sum  Orientation=up  Inputs=+|-
  Sum5 : Sum  Orientation=left  Inputs=++|
  Sum6 : Sum  Orientation=left  Inputs=|++
  attrito albero motore : Gain  Orientation=down  Gain=bm
  attrito albero motore1 : Gain  Orientation=down  Gain=p
  bTw (w->b) : Subsystem  Orientation=left
  bTw' (b->w) : Subsystem
  sTt (t->s) : Gain  Orientation=left  Gain=sTt  Multiplication=Matrix(K*u) (u vector)
  sTt' (s->t) : Gain  Gain=sTt'  Multiplication=Matrix(K*u) (u vector)
  tTb (b->t) : Gain  Orientation=left  Gain=tTb  Multiplication=Matrix(K*u) (u vector)
  tTb' (t->b) : Gain  Gain=tTb'  Multiplication=Matrix(K*u) (u vector)
  Is : Outport  Orientation=left
  m : Outport  Orientation=down  Port=2
  Wm : Outport  Port=3
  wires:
  Fwe/1(E_f) -> Sum6/2
  Sum6/1 -> Sum3/1  "0"
  Bus Creator/1 -> m/1
  tTb (b->t)/1 -> Bus Creator/4, sTt (t->s)/1  "Currents It"
  Te/1 -> Bus Creator/12, Sum5/2  "Torque Te"
  Vs/1 -> Bus Creator/1, sTt' (s->t)/1  "Voltages Vs"
  bTw (w->b)/1(Ib) -> Bus Creator/6, tTb (b->t)/1  "Currents Ib"
  bTw' (b->w)/1(Vw) -> Bus Creator/7, Sum1/1  "Voltages Vw"
  attrito albero motore/1 -> Sum5/1
  Motor inertia/1 -> Bus Creator/11, Kw_e'/1(Wm), attrito albero motore/1, Wm/1, attrito albero motore1/1  "Velocity Wm"
  Integrator4/1 -> Motor inertia/1
  Sum4/1 -> Integrator4/1
  Kw_e'/1(Ew) -> Bus Creator/9, Sum6/1  "Back EMF Ew"
  Kw_e/1(Tm) -> Bus Creator/10, Sum4/1  "Torque Tm"
  Owe/1(E_o) -> Sum3/2
  1/Lwe/1 -> bTw (w->b)/1(Iw), Bus Creator/8, Fwe/1(Iw), Kw_e/1(Iw), Owe/1(Iw), Rwe/1  "Currents Iw"
  Integrator3/1 -> 1/Lwe/1
  Sum1/1 -> Integrator3/1
  Integrator2/1 -> Bus Creator/14, [th_e]  "AngleThe"
  attrito albero motore1/1 -> Bus Creator/13, [w_e], Integrator2/1  "Velocity We"
  tTb' (t->b)/1 -> Bus Creator/5, bTw' (b->w)/1(Vb)  "Voltages Vb"
  Sum5/1 -> Sum4/2
  ws/1 -> [w_s]
  Rwe/1 -> Sum2/2
  Sum3/1 -> Sum2/1
  Sum2/1 -> Sum1/2
  sTt (t->s)/1 -> Bus Creator/2, Is/1  "Currents Is"
  sTt' (s->t)/1 -> Bus Creator/3, tTb' (t->b)/1  "Voltages Vt"

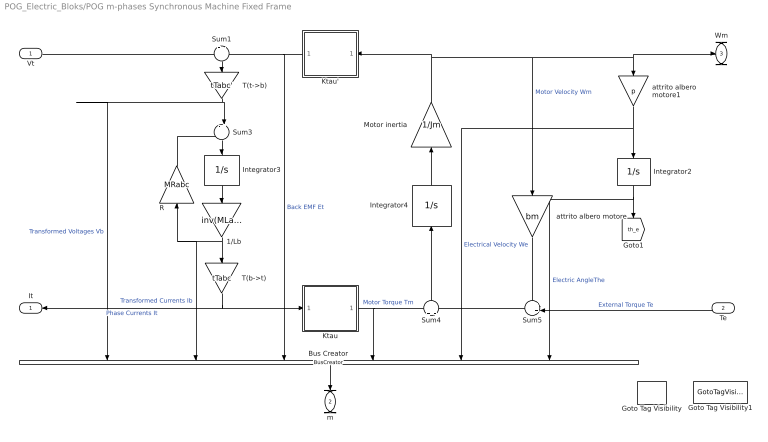
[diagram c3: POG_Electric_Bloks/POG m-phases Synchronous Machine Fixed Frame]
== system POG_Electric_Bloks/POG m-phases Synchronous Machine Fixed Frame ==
  Vt : Inport
  Te : Inport  Orientation=left  Port=2
  1/Lb : Gain  Orientation=down  Gain=inv(MLabc)  Multiplication=Matrix(K*u) (u vector)
  Bus Creator : BusCreator  Orientation=down  Inputs=6
  Goto Tag Visibility : GotoTagVisibility
  Goto Tag Visibility1 : GotoTagVisibility
  Integrator2 : Integrator  Orientation=down  InitialCondition=Thm0*p
  Integrator3 : Integrator  Orientation=down  InitialCondition=Ibt0
  Integrator4 : Integrator  Orientation=up  InitialCondition=Wm0*Jm
  Ktau : Subsystem
  Ktau' : Subsystem  Orientation=left
  Motor inertia : Gain  Orientation=up  Gain=1/Jm
  R : Gain  Orientation=up  Gain=MRabc  Multiplication=Matrix(K*u) (u vector)
  Sum1 : Sum  Orientation=down  Inputs=+|-
  Sum3 : Sum  Orientation=down  Inputs=-+|
  Sum4 : Sum  Orientation=up  Inputs=+|-
  Sum5 : Sum  Orientation=left  Inputs=++|
  T(b->t) : Gain  Orientation=down  Gain=tTabc  Multiplication=Matrix(K*u) (u vector)
  T(t->b) : Gain  Orientation=down  Gain=tTabc'  Multiplication=Matrix(K*u) (u vector)
  attrito albero motore : Gain  Orientation=down  Gain=bm
  attrito albero motore1 : Gain  Orientation=down  Gain=p
  It : Outport  Orientation=left
  m : Outport  Orientation=down  Port=2
  Wm : Outport  Port=3
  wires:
  Sum5/1 -> Sum4/2
  attrito albero motore1/1 -> Integrator2/1, Bus Creator/5  "Electrical Velocity We"
  Integrator2/1 -> [th_e], Bus Creator/6  "Electric AngleThe"
  Ktau/1(Tm) -> Sum4/1, Bus Creator/4  "Motor Torque Tm"
  Sum4/1 -> Integrator4/1
  Integrator4/1 -> Motor inertia/1
  Motor inertia/1 -> Ktau'/1(Wm), attrito albero motore/1, attrito albero motore1/1, Wm/1  "Motor Velocity Wm"
  attrito albero motore/1 -> Sum5/1
  Te/1 -> Sum5/2  "External Torque Te"
  Bus Creator/1 -> m/1
  Integrator3/1 -> 1/Lb/1
  1/Lb/1 -> T(b->t)/1, R/1, Bus Creator/2  "Transformed Currents Ib"
  Sum3/1 -> Integrator3/1
  Sum1/1 -> T(t->b)/1
  Vt/1 -> Sum1/1
  T(b->t)/1 -> It/1, Ktau/1(It)  "Phase Currents It"
  Ktau'/1(Et) -> Sum1/2, Bus Creator/3  "Back EMF Et"
  R/1 -> Sum3/1
  T(t->b)/1 -> Sum3/2, Bus Creator/1  "Transformed Voltages Vb"

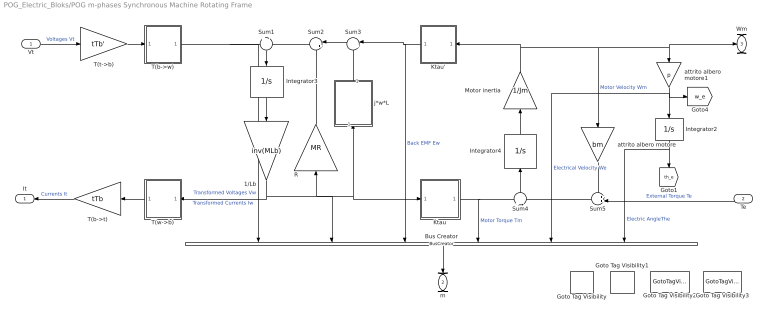
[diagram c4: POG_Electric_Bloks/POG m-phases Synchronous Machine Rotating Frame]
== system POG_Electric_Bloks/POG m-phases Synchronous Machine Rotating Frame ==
  Vt : Inport
  Te : Inport  Orientation=left  Port=2
  1/Lb : Gain  Orientation=down  Gain=inv(MLb)  Multiplication=Matrix(K*u) (u vector)
  Bus Creator : BusCreator  Orientation=down  Inputs=6
  Goto Tag Visibility{,1..3} (4 alike) : GotoTagVisibility
  Integrator2 : Integrator  Orientation=down  InitialCondition=Thm0*p
  Integrator3 : Integrator  Orientation=down  InitialCondition=MLb*Iw0
  Integrator4 : Integrator  Orientation=up  InitialCondition=Wm0*Jm
  Ktau : Subsystem
  Ktau' : Subsystem  Orientation=left
  Motor inertia : Gain  Orientation=up  Gain=1/Jm
  R : Gain  Orientation=up  Gain=MR  Multiplication=Matrix(K*u) (u vector)
  Sum1 : Sum  Orientation=down  Inputs=+|-
  Sum2 : Sum  Orientation=left  Inputs=|++
  Sum3 : Sum  Orientation=left  Inputs=|++
  Sum4 : Sum  Orientation=up  Inputs=+|-
  Sum5 : Sum  Orientation=left  Inputs=++|
  T(b->t) : Gain  Orientation=left  Gain=tTb  Multiplication=Matrix(K*u) (u vector)
  T(b->w) : Subsystem
  T(t->b) : Gain  Gain=tTb'  Multiplication=Matrix(K*u) (u vector)
  T(w->b) : Subsystem  Orientation=left
  attrito albero motore : Gain  Orientation=down  Gain=bm
  attrito albero motore1 : Gain  Orientation=down  Gain=p
  j*w*L : Subsystem  Orientation=up
  It : Outport  Orientation=left
  m : Outport  Orientation=down  Port=2
  Wm : Outport  Port=3
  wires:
  Bus Creator/1 -> m/1
  T(b->t)/1 -> It/1  "Currents It"
  Te/1 -> Sum5/2  "External Torque Te"
  Vt/1 -> T(t->b)/1  "Voltages Vt"
  T(w->b)/1(It) -> T(b->t)/1
  T(b->w)/1(Vw) -> Bus Creator/1, Sum1/1  "Transformed Voltages Vw"
  attrito albero motore/1 -> Sum5/1
  Motor inertia/1 -> Ktau'/1(Wm), Wm/1, attrito albero motore1/1, attrito albero motore/1  "Motor Velocity Wm"
  Integrator4/1 -> Motor inertia/1
  Sum4/1 -> Integrator4/1
  Ktau'/1(Ew) -> Bus Creator/3, Sum3/1  "Back EMF Ew"
  Ktau/1(Tm) -> Bus Creator/4, Sum4/1  "Motor Torque Tm"
  j*w*L/1(Out1) -> Sum3/2
  Sum3/1 -> Sum2/1
  R/1 -> Sum2/2
  Sum2/1 -> Sum1/2
  1/Lb/1 -> Bus Creator/2, Ktau/1(Iw), j*w*L/1(In1), R/1, T(w->b)/1(Iw)  "Transformed Currents Iw"
  Integrator3/1 -> 1/Lb/1
  Sum1/1 -> Integrator3/1
  Integrator2/1 -> Bus Creator/6, [th_e]  "Electric AngleThe"
  attrito albero motore1/1 -> [w_e], Integrator2/1, Bus Creator/5  "Electrical Velocity We"
  T(t->b)/1 -> T(b->w)/1(Vt)
  Sum5/1 -> Sum4/2

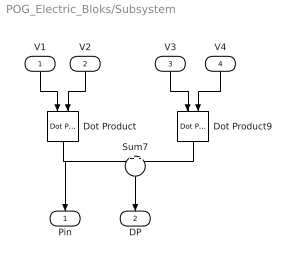
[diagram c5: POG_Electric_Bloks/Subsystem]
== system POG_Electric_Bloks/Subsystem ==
  V1 : Inport  Orientation=down
  V2 : Inport  Orientation=down  Port=2
  V3 : Inport  Orientation=down  Port=3
  V4 : Inport  Orientation=down  Port=4
  Dot Product : simulink/Math Operations/Dot Product  Orientation=down  InputSameDT=on  OutDataType=sfix(16)  OutScaling=2^-10  DoSatur=off
  Dot Product9 : simulink/Math Operations/Dot Product  Orientation=down  InputSameDT=on  OutDataType=sfix(16)  OutScaling=2^-10  DoSatur=off
  Sum7 : Sum  Orientation=down  Inputs=+|-
  Pin : Outport  Orientation=down
  DP : Outport  Orientation=down  Port=2
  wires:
  Sum7/1 -> DP/1
  V4/1 -> Dot Product9/2
  V3/1 -> Dot Product9/1
  V2/1 -> Dot Product/2
  V1/1 -> Dot Product/1
  Dot Product9/1 -> Sum7/2
  Dot Product/1 -> Pin/1, Sum7/1

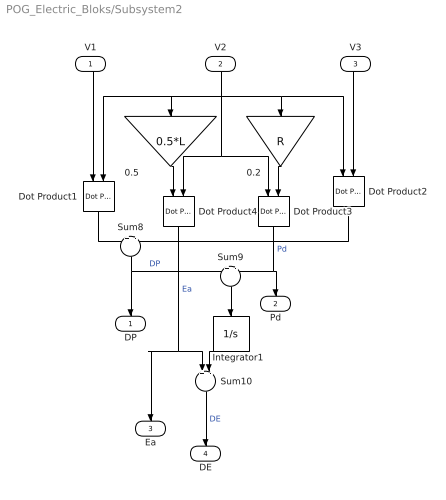
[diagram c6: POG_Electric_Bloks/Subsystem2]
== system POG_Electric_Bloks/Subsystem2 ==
  V1 : Inport  Orientation=down
  V2 : Inport  Orientation=down  Port=2
  V3 : Inport  Orientation=down  Port=3
  0.2 : Gain  Orientation=down  Gain=R  Multiplication=Matrix(K*u)
  0.5 : Gain  Orientation=down  Gain=0.5*L  Multiplication=Matrix(K*u)
  Dot Product{1..4} (4 alike) : simulink/Math Operations/Dot Product  Orientation=down  InputSameDT=on  OutDataType=sfix(16)  OutScaling=2^-10  DoSatur=off
  Integrator1 : Integrator  Orientation=down
  Sum10 : Sum  Orientation=down  Inputs=+|-
  Sum8 : Sum  Orientation=down  Inputs=+|-
  Sum9 : Sum  Orientation=down  Inputs=+|-
  DP : Outport  Orientation=down
  Pd : Outport  Orientation=down  Port=2
  Ea : Outport  Orientation=down  Port=3
  DE : Outport  Orientation=down  Port=4
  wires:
  0.2/1 -> Dot Product3/2
  Sum10/1 -> DE/1  "DE"
  V1/1 -> Dot Product1/1
  V3/1 -> Dot Product2/2
  V2/1 -> Dot Product1/2, Dot Product3/1, Dot Product4/2, 0.2/1, Dot Product2/1, 0.5/1
  Integrator1/1 -> Sum10/2
  Dot Product4/1 -> Sum10/1, Ea/1  "Ea"
  0.5/1 -> Dot Product4/1
  Dot Product3/1 -> Pd/1, Sum9/2  "Pd"
  Sum9/1 -> Integrator1/1
  Dot Product2/1 -> Sum8/2
  Sum8/1 -> DP/1, Sum9/1  "DP"
  Dot Product1/1 -> Sum8/1

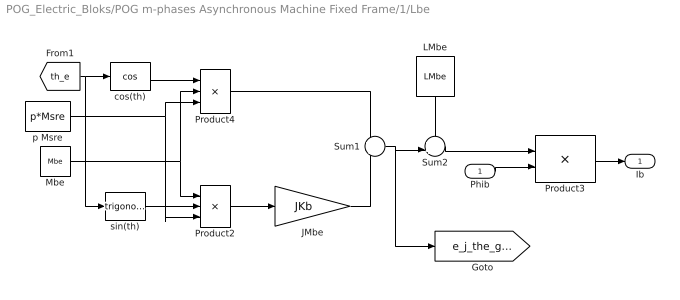
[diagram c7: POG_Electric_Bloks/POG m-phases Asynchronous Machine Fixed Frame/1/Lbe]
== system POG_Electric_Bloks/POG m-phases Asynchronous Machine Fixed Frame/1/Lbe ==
  Phib : Inport
  JMbe : Gain  Gain=JKb  Multiplication=Matrix(K*u)
  LMbe : Constant  Orientation=down  Value=LMbe  VectorParams1D=off
  Mbe : Constant  Value=Mbe
  Product2 : Product  Inputs=3
  Product3 : Product  Inputs=/*  Multiplication=Matrix(*)
  Product4 : Product  Inputs=3
  Sum1 : Sum  Inputs=+|-
  Sum2 : Sum  Inputs=++|
  cos(th) : Trigonometry  Operator=cos
  p Msre : Constant  Value=p*Msre
  sin(th) : Trigonometry
  Ib : Outport
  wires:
  Sum2/1 -> Product3/1
  Sum1/1 -> [e_j_the_goto], Sum2/2
  LMbe/1 -> Sum2/1
  JMbe/1 -> Sum1/2
  Product4/1 -> Sum1/1
  Product2/1 -> JMbe/1
  p Msre/1 -> Product2/3, Product4/3
  sin(th)/1 -> Product2/2
  cos(th)/1 -> Product4/1
  [th_e] -> sin(th)/1, cos(th)/1
  Mbe/1 -> Product2/1, Product4/2
  Phib/1 -> Product3/2
  Product3/1 -> Ib/1

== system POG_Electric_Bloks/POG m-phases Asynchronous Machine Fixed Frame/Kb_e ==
  Ib : Inport
  Dot Product : simulink/Math Operations/Dot Product  InputSameDT=on  OutDataType=sfix(16)  OutScaling=2^-10  DoSatur=off
  JKe : Gain  Gain=p*JKb/2  Multiplication=Matrix(K*u) (u vector)
  Product3 : Product  Multiplication=Matrix(*)
  Tm : Outport
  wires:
  Product3/1 -> [Ktau_goto], Dot Product/1
  JKe/1 -> Product3/2
  [e_j_the_goto] -> Product3/1
  Ib/1 -> Dot Product/2, JKe/1
  Dot Product/1 -> Tm/1

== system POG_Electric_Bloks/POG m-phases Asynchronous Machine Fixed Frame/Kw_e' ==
  Wm : Inport
  Product : Product  Multiplication=Matrix(*)
  Eb : Outport
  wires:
  [Ktau_goto] -> Product/1
  Product/1 -> Eb/1
  Wm/1 -> Product/2

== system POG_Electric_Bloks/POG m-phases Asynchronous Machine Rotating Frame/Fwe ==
  Iw : Inport
  JFe : Constant  Value=JFe
  Product : Product  Multiplication=Matrix(*)
  Product1 : Product
  E_f : Outport
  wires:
  JFe/1 -> Product1/2
  [w_e] -> Product1/1
  Iw/1 -> Product/2
  Product/1 -> E_f/1
  Product1/1 -> Product/1

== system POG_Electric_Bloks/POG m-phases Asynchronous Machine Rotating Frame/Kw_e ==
  Iw : Inport
  Dot Product : simulink/Math Operations/Dot Product  InputSameDT=on  OutDataType=sfix(16)  OutScaling=2^-10  DoSatur=off
  JKe : Gain  Gain=JKe  Multiplication=Matrix(K*u) (u vector)
  Tm : Outport
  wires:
  JKe/1 -> [Ktau_goto], Dot Product/1
  Iw/1 -> Dot Product/2, JKe/1
  Dot Product/1 -> Tm/1

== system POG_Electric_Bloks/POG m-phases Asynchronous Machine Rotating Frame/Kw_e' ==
  Wm : Inport
  Product : Product  Multiplication=Matrix(*)
  Ew : Outport
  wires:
  [Ktau_goto] -> Product/1
  Product/1 -> Ew/1
  Wm/1 -> Product/2

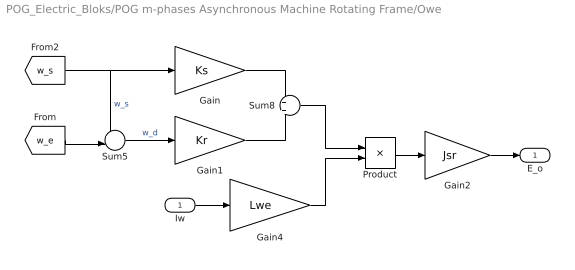
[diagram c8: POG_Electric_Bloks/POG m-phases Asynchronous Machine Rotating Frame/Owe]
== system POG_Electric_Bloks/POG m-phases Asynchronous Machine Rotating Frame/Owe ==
  Iw : Inport
  Gain : Gain  Gain=Ks  Multiplication=Matrix(K*u) (u vector)
  Gain1 : Gain  Gain=Kr  Multiplication=Matrix(K*u) (u vector)
  Gain2 : Gain  Gain=Jsr  Multiplication=Matrix(K*u) (u vector)
  Gain4 : Gain  Gain=Lwe  Multiplication=Matrix(K*u) (u vector)
  Product : Product
  Sum5 : Sum  Inputs=+-|
  Sum8 : Sum  Inputs=+|+
  E_o : Outport
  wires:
  Gain2/1 -> E_o/1
  Product/1 -> Gain2/1
  Gain4/1 -> Product/2
  Sum8/1 -> Product/1
  Iw/1 -> Gain4/1
  Sum5/1 -> Gain1/1  "w_d"
  [w_e] -> Sum5/2
  [w_s] -> Sum5/1, Gain/1  "w_s"
  Gain/1 -> Sum8/1
  Gain1/1 -> Sum8/2

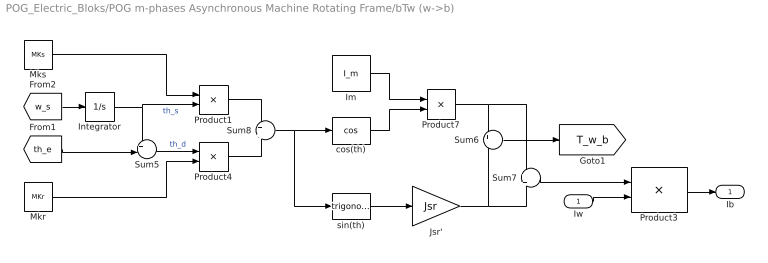
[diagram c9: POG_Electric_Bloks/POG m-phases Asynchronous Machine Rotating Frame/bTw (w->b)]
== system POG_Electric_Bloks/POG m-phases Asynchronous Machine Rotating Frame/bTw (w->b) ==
  Iw : Inport
  Im : Constant  Value=I_m  VectorParams1D=off
  Integrator : Integrator
  Jsr' : Gain  Gain=Jsr  Multiplication=Matrix(K*u)
  Mkr : Constant  Value=MKr
  Mks : Constant  Value=MKs
  Product1 : Product
  Product3 : Product  Multiplication=Matrix(*)
  Product4 : Product
  Product7 : Product
  Sum5 : Sum  Inputs=+-|
  Sum6 : Sum  Inputs=+|-
  Sum7 : Sum  Inputs=+|+
  Sum8 : Sum  Inputs=+|+
  cos(th) : Trigonometry  Operator=cos
  sin(th) : Trigonometry
  Ib : Outport
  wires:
  Sum5/1 -> Product4/1  "th_d"
  [th_e] -> Sum5/2
  Mkr/1 -> Product4/2
  [w_s] -> Integrator/1
  Integrator/1 -> Sum5/1, Product1/2  "th_s"
  Sum6/1 -> [T_w_b]
  sin(th)/1 -> Jsr'/1
  Sum8/1 -> cos(th)/1, sin(th)/1
  cos(th)/1 -> Product7/2
  Im/1 -> Product7/1
  Product7/1 -> Sum6/1, Sum7/1
  Jsr'/1 -> Sum6/2, Sum7/2
  Iw/1 -> Product3/2
  Product3/1 -> Ib/1
  Sum7/1 -> Product3/1
  Mks/1 -> Product1/1
  Product1/1 -> Sum8/1
  Product4/1 -> Sum8/2

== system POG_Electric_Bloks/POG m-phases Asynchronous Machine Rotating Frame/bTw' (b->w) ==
  Vb : Inport
  Product : Product  Multiplication=Matrix(*)
  Vw : Outport
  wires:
  [T_w_b] -> Product/1
  Product/1 -> Vw/1
  Vb/1 -> Product/2

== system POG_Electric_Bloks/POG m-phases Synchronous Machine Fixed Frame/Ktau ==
  It : Inport
  Constant : Constant  Value=Sfasa  VectorParams1D=off
  Dot Product : simulink/Math Operations/Dot Product  InputSameDT=on  OutDataType=sfix(16)  OutScaling=2^-10  DoSatur=off
  Lookup Table : Lookup  InputValues=LkUpT_in  OutputValues=LkUpT_out
  MATLAB Fcn1 : MATLABFcn  MATLABFcn=rem(u,2*pi)
  Sum1 : Sum  Inputs=|++
  Tm : Outport
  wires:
  Dot Product/1 -> Tm/1
  It/1 -> Dot Product/2
  Lookup Table/1 -> Dot Product/1, [Ktau_goto]
  MATLAB Fcn1/1 -> Lookup Table/1
  [th_e] -> Sum1/1
  Sum1/1 -> MATLAB Fcn1/1
  Constant/1 -> Sum1/2

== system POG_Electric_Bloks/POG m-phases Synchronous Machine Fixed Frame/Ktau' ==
  Wm : Inport
  Product : Product  Multiplication=Matrix(*)
  Et : Outport
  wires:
  Wm/1 -> Product/2
  Product/1 -> Et/1
  [Ktau_goto] -> Product/1
